| TEXAS INSTRUMENTS INCORPORATED
| Standard Linear and Logic Group
| IBIS Model of SN74LVCH16244A
| 16 Bit Buffer/Driver With 3 State Outputs
| This file contains package information for the following:
|  TSSOP 48-pin (DGG) package as [Component] LVCH16244A_DGG
|  SSOP 48-pin (DL) package as [Component] LVCH16244A_DL
| This device can be powered at the following Vccs:
|  3.3 volt Vcc
|  2.5 volt Vcc
|  1.8 volt Vcc
| This file provides unique models under the [Model Selector] for each Vcc.
| For operation at a specific Vcc, select the appropriate model after each
| [Model Selector] keyword.
[IBIS Ver]   3.2
[Comment char]  |_char
[File Name]   sn74lvch16244a.ibs
[File Rev]   1.1 | e_die
[Date]   March 8, 2002
[Source]   Data created from TI-SPICE simulations at TI-SLL.
[Notes]   The following is an IBIS list for the LVCH16244A.
   Please contact sllibis@ti.com with questions and
   comments concerning SLL IBIS models.
   - As there is no power clamp diode in the Input and I/O
   Models, we removed the Pwr Clamp table data from those Models.
   - Due to BUS-HOLD Circuit, there are non-monotonic
   warnings in I/O GND Clamp curve.
   -Due to the fact that the Device is 5-V Input/Output
   tolarent, the output model has some Non-Monotonic Warnings.
   - C_comp values are taken at a different test condition than
   the data sheet.
[Disclaimer] Property of Texas Instruments Incorporated.  Unauthorized
   reproduction and/or distribution is strictly prohibited.
   This product is protected under copyright law.
   Created  2001, (C) Copyright  2001, Texas Instruments
   Incorporated, All Rights Reserved
   UNLESS THERE IS A SIGNED, WRITTEN AGREEMENT TO THE
   CONTRARY, TEXAS INSTRUMENTS (TI) IS PROVIDING THE IBIS
   MODELS  AND WITHOUT ANY WARRANTY, EXPRESSED OR
   IMPLIED.  TI assumes no liability for:
   1) the accuracy of the IBIS models provided to your
   company;
   2) the proper functioning of these IBIS Models in your
   design or for any resulting applications; or
   3) infringement of patents, copyrights or intellectual
   property rights resulting from your use of these IBIS
   models.
   TI provides IBIS Models as a service to our customers.
   You and your company shall not distribute, sell or give
   these models to anyone else without prior written
   permission from TI.
   TI reserves the right to make changes to our products or
   to discontinue any semiconductor product or service
   without notice, and advises our customers to obtain the
   latest version of relevant information to verify, before
   placing orders, that the information being relied on is
   current.
   Please be aware that your receipt and use of the IBIS
   information provided shall serve as acceptance of these
   terms and conditions.  If you do not accept these terms,
   you should return or destroy the IBIS models and any
   other accompanying information immediately.
| Component LVCH16244A_DGG 48-pin TSSOP
[Component]   LVCH16244A_DGG
[Manufacturer]   Texas Instruments, Inc.
[Package]
|   typ   min   max
R_pkg   6.200e-02   5.000e-02   7.800e-02
L_pkg   3.527e-09   3.128e-09   4.255e-09
C_pkg   5.300e-13   4.170e-13   6.850e-13
[Pin]   signal_name   model_name   R_pin   L_pin   C_pin
1   1OE   LVCH16244A_OEIN   5.000e-02   4.250e-09   6.710e-13
2   1Y1   LVCH16244A_OUT   5.700e-02   3.956e-09   6.740e-13
3   1Y2   LVCH16244A_OUT   7.100e-02   3.922e-09   6.190e-13
4   GND   GND   7.800e-02   3.841e-09   6.180e-13
5   1Y3   LVCH16244A_OUT   5.600e-02   3.535e-09   5.550e-13
6   1Y4   LVCH16244A_OUT   5.800e-02   3.464e-09   5.030e-13
7   VCC   POWER   6.000e-02   3.362e-09   4.980e-13
8   2Y1   LVCH16244A_OUT   6.100e-02   3.293e-09   4.620e-13
9   2Y2   LVCH16244A_OUT   6.300e-02   3.240e-09   4.550e-13
10   GND   GND   6.300e-02   3.175e-09   4.420e-13
11   2Y3   LVCH16244A_OUT   6.400e-02   3.153e-09   4.290e-13
12   2Y4   LVCH16244A_OUT   6.500e-02   3.128e-09   4.180e-13
13   3Y1   LVCH16244A_OUT   6.500e-02   3.128e-09   4.180e-13
14   3Y2   LVCH16244A_OUT   6.400e-02   3.154e-09   4.290e-13
15   GND   GND   6.300e-02   3.174e-09   4.420e-13
16   3Y3   LVCH16244A_OUT   6.300e-02   3.241e-09   4.550e-13
17   3Y4   LVCH16244A_OUT   6.100e-02   3.293e-09   4.620e-13
18   VCC   POWER   6.000e-02   3.362e-09   4.970e-13
19   4Y1   LVCH16244A_OUT   5.800e-02   3.464e-09   5.030e-13
20   4Y2   LVCH16244A_OUT   5.600e-02   3.537e-09   5.600e-13
21   GND   GND   7.700e-02   3.839e-09   6.260e-13
22   4Y3   LVCH16244A_OUT   7.100e-02   3.917e-09   6.270e-13
23   4Y4   LVCH16244A_OUT   5.800e-02   3.955e-09   6.850e-13
24   4OE   LVCH16244A_OEIN   5.200e-02   4.255e-09   6.790e-13
25   3OE   LVCH16244A_OEIN   5.100e-02   4.254e-09   6.760e-13
26   4A4   LVCH16244A_IN   5.800e-02   3.957e-09   6.790e-13
27   4A3   LVCH16244A_IN   7.100e-02   3.920e-09   6.210e-13
28   GND   GND   7.800e-02   3.843e-09   6.220e-13
29   4A2   LVCH16244A_IN   5.600e-02   3.539e-09   5.600e-13
30   4A1   LVCH16244A_IN   5.800e-02   3.466e-09   5.030e-13
31   VCC   POWER   6.000e-02   3.363e-09   4.970e-13
32   3A4   LVCH16244A_IN   6.100e-02   3.294e-09   4.620e-13
33   3A3   LVCH16244A_IN   6.300e-02   3.241e-09   4.540e-13
34   GND   GND   6.300e-02   3.175e-09   4.410e-13
35   3A2   LVCH16244A_IN   6.400e-02   3.153e-09   4.290e-13
36   3A1   LVCH16244A_IN   6.500e-02   3.129e-09   4.170e-13
37   2A4   LVCH16244A_IN   6.500e-02   3.129e-09   4.170e-13
38   2A3   LVCH16244A_IN   6.400e-02   3.152e-09   4.290e-13
39   GND   GND   6.400e-02   3.176e-09   4.410e-13
40   2A2   LVCH16244A_IN   6.300e-02   3.241e-09   4.540e-13
41   2A1   LVCH16244A_IN   6.100e-02   3.293e-09   4.620e-13
42   VCC   POWER   6.000e-02   3.363e-09   4.970e-13
43   1A4   LVCH16244A_IN   5.800e-02   3.464e-09   5.030e-13
44   1A3   LVCH16244A_IN   5.600e-02   3.534e-09   5.610e-13
45   GND   GND   7.800e-02   3.841e-09   6.260e-13
46   1A2   LVCH16244A_IN   7.100e-02   3.920e-09   6.220e-13
47   1A1   LVCH16244A_IN   5.700e-02   3.955e-09   6.770e-13
48   2OE   LVCH16244A_OEIN   5.100e-02   4.252e-09   6.720e-13
| Component LVCH16244A_DL 48-pin SSOP
[Component]   LVCH16244A_DL
[Manufacturer]   Texas Instruments, Inc.
[Package]
|   typ   min   max
R_pkg   4.800e-02   3.800e-02   5.300e-02
L_pkg   6.046e-09   5.084e-09   7.968e-09
C_pkg   8.130e-13   5.690e-13   1.157e-12
[Pin]   signal_name   model_name   R_pin   L_pin   C_pin
1   1OE   LVCH16244A_OEIN   4.600e-02   7.968e-09   1.017e-12
2   1Y1   LVCH16244A_OUT   4.400e-02   7.299e-09   1.157e-12
3   1Y2   LVCH16244A_OUT   4.300e-02   6.765e-09   1.058e-12
4   GND   GND   4.100e-02   6.269e-09   9.330e-13
5   1Y3   LVCH16244A_OUT   3.800e-02   5.856e-09   8.290e-13
6   1Y4   LVCH16244A_OUT   4.600e-02   5.802e-09   7.900e-13
7   VCC   POWER   5.000e-02   5.656e-09   7.380e-13
8   2Y1   LVCH16244A_OUT   5.300e-02   5.500e-09   6.430e-13
9   2Y2   LVCH16244A_OUT   5.200e-02   5.304e-09   6.060e-13
10   GND   GND   5.300e-02   5.189e-09   5.830e-13
11   2Y3   LVCH16244A_OUT   5.100e-02   5.084e-09   5.690e-13
12   2Y4   LVCH16244A_OUT   5.300e-02   5.862e-09   8.330e-13
13   3Y1   LVCH16244A_OUT   5.300e-02   5.862e-09   8.330e-13
14   3Y2   LVCH16244A_OUT   5.100e-02   5.084e-09   5.690e-13
15   GND   GND   5.300e-02   5.189e-09   5.830e-13
16   3Y3   LVCH16244A_OUT   5.200e-02   5.304e-09   6.060e-13
17   3Y4   LVCH16244A_OUT   5.300e-02   5.500e-09   6.430e-13
18   VCC   POWER   5.000e-02   5.656e-09   7.380e-13
19   4Y1   LVCH16244A_OUT   4.600e-02   5.802e-09   7.900e-13
20   4Y2   LVCH16244A_OUT   3.800e-02   5.856e-09   8.290e-13
21   GND   GND   4.100e-02   6.269e-09   9.330e-13
22   4Y3   LVCH16244A_OUT   4.300e-02   6.765e-09   1.058e-12
23   4Y4   LVCH16244A_OUT   4.400e-02   7.299e-09   1.157e-12
24   4OE   LVCH16244A_OEIN   4.600e-02   7.968e-09   1.017e-12
25   3OE   LVCH16244A_OEIN   4.600e-02   7.968e-09   1.017e-12
26   4A4   LVCH16244A_IN   4.400e-02   7.299e-09   1.157e-12
27   4A3   LVCH16244A_IN   4.300e-02   6.765e-09   1.058e-12
28   GND   GND   4.100e-02   6.269e-09   9.330e-13
29   4A2   LVCH16244A_IN   3.800e-02   5.856e-09   8.290e-13
30   4A1   LVCH16244A_IN   4.600e-02   5.802e-09   7.900e-13
31   VCC   POWER   5.000e-02   5.656e-09   7.380e-13
32   3A4   LVCH16244A_IN   5.300e-02   5.500e-09   6.430e-13
33   3A3   LVCH16244A_IN   5.200e-02   5.304e-09   6.060e-13
34   GND   GND   5.300e-02   5.189e-09   5.830e-13
35   3A2   LVCH16244A_IN   5.100e-02   5.084e-09   5.690e-13
36   3A1   LVCH16244A_IN   5.300e-02   5.862e-09   8.330e-13
37   2A4   LVCH16244A_IN   5.300e-02   5.862e-09   8.330e-13
38   2A3   LVCH16244A_IN   5.100e-02   5.084e-09   5.690e-13
39   GND   GND   5.300e-02   5.189e-09   5.830e-13
40   2A2   LVCH16244A_IN   5.200e-02   5.304e-09   6.060e-13
41   2A1   LVCH16244A_IN   5.300e-02   5.500e-09   6.430e-13
42   VCC   POWER   5.000e-02   5.656e-09   7.380e-13
43   1A4   LVCH16244A_IN   4.600e-02   5.802e-09   7.900e-13
44   1A3   LVCH16244A_IN   3.800e-02   5.856e-09   8.290e-13
45   GND   GND   4.100e-02   6.269e-09   9.330e-13
46   1A2   LVCH16244A_IN   4.300e-02   6.765e-09   1.058e-12
47   1A1   LVCH16244A_IN   4.400e-02   7.299e-09   1.157e-12
48   2OE   LVCH16244A_OEIN   4.600e-02   7.967e-09   1.017e-12
|   Component   LVCH16244A_DGV   48-pin   TVSOP
[Component]   LVCH16244A_DGV
[Manufacturer]   Texas   Instruments,   Inc.
[Package]
|   typ   min   max
R_pkg   0.07   0.049   0.085
L_pkg   3.01E-09   2.74E-09   3.41E-09
C_pkg   3.71E-13   2.94E-13   5.11E-13
[Pin]   signal_name   model_name   R_pin   L_pin   C_pin
1   1OE   LVCH16244A_OEIN   0.049   3.39E-09   4.97E-13
2   1Y1   LVCH16244A_OUT   0.06   3.25E-09   5.02E-13
3   1Y2   LVCH16244A_OUT   0.077   3.31E-09   4.51E-13
4   GND   GND   0.085   3.3E-09   4.04E-13
5   1Y3   LVCH16244A_OUT   0.083   3.14E-09   3.6E-13
6   1Y4   LVCH16244A_OUT   0.077   3.02E-09   3.63E-13
7   VCC   POWER   0.065   2.88E-09   3.49E-13
8   2Y1   LVCH16244A_OUT   0.066   2.83E-09   3.14E-13
9   2Y2   LVCH16244A_OUT   0.067   2.8E-09   3.14E-13
10   GND   GND   0.069   2.75E-09   3.08E-13
11   2Y3   LVCH16244A_OUT   0.07   2.75E-09   3.01E-13
12   2Y4   LVCH16244A_OUT   0.071   2.75E-09   2.94E-13
13   3Y1   LVCH16244A_OUT   0.07   2.74E-09   2.94E-13
14   3Y2   LVCH16244A_OUT   0.07   2.75E-09   3.01E-13
15   GND   GND   0.069   2.75E-09   3.08E-13
16   3Y3   LVCH16244A_OUT   0.067   2.8E-09   3.14E-13
17   3Y4   LVCH16244A_OUT   0.066   2.83E-09   3.14E-13
18   VCC   POWER   0.065   2.88E-09   3.5E-13
19   4Y1   LVCH16244A_OUT   0.075   3.01E-09   3.63E-13
20   4Y2   LVCH16244A_OUT   0.08   3.13E-09   3.58E-13
21   GND   GND   0.084   3.3E-09   4.03E-13
22   4Y3   LVCH16244A_OUT   0.078   3.31E-09   4.52E-13
23   4Y4   LVCH16244A_OUT   0.062   3.26E-09   5.01E-13
24   4OE   LVCH16244A_OEIN   0.052   3.4E-09   4.96E-13
25   3OE   LVCH16244A_OEIN   0.053   3.4E-09   5.05E-13
26   4A4   LVCH16244A_IN   0.062   3.25E-09   5.11E-13
27   4A3   LVCH16244A_IN   0.077   3.31E-09   4.53E-13
28   GND   GND   0.082   3.29E-09   4.03E-13
29   4A2   LVCH16244A_IN   0.078   3.12E-09   3.59E-13
30   4A1   LVCH16244A_IN   0.074   3.01E-09   3.63E-13
31   VCC   POWER   0.065   2.88E-09   3.49E-13
32   3A4   LVCH16244A_IN   0.067   2.83E-09   3.14E-13
33   3A3   LVCH16244A_IN   0.067   2.8E-09   3.14E-13
34   GND   GND   0.069   2.75E-09   3.07E-13
35   3A2   LVCH16244A_IN   0.07   2.75E-09   3.01E-13
36   3A1   LVCH16244A_IN   0.07   2.74E-09   2.94E-13
37   2A4   LVCH16244A_IN   0.07   2.74E-09   2.94E-13
38   2A3   LVCH16244A_IN   0.07   2.75E-09   3.01E-13
39   GND   GND   0.069   2.75E-09   3.07E-13
40   2A2   LVCH16244A_IN   0.068   2.8E-09   3.14E-13
41   2A1   LVCH16244A_IN   0.067   2.83E-09   3.14E-13
42   VCC   POWER   0.064   2.88E-09   3.49E-13
43   1A4   LVCH16244A_IN   0.072   3E-09   3.62E-13
44   1A3   LVCH16244A_IN   0.078   3.12E-09   3.59E-13
45   GND   GND   0.084   3.3E-09   4.03E-13
46   1A2   LVCH16244A_IN   0.077   3.31E-09   4.51E-13
47   1A1   LVCH16244A_IN   0.062   3.26E-09   4.99E-13
48   2OE   LVCH16244A_OEIN   0.053   3.41E-09   4.94E-13
| Model LVCH16244A_IN
[Model Selector]   LVCH16244A_IN
LVCH16244A_IN_33   3.3 volt Vcc
LVCH16244A_IN_25   2.5 volt Vcc
LVCH16244A_IN_18   1.8 volt Vcc
| Model LVCH16244A_OEIN
[Model Selector]   LVCH16244A_OEIN
LVCH16244A_OEIN_33   3.3 volt Vcc
LVCH16244A_OEIN_25   2.5 volt Vcc
LVCH16244A_OEIN_18   1.8 volt Vcc
| Model LVCH16244A_OUT
[Model Selector]   LVCH16244A_OUT
LVCH16244A_OUT_33   3.3 volt Vcc
LVCH16244A_OUT_25   2.5 volt Vcc
LVCH16244A_OUT_18   1.8 volt Vcc
| Models and submodels in the file (9): LVCH16244A_IN_33 (Input), LVCH16244A_IN_25 (Input), LVCH16244A_IN_18 (Input), LVCH16244A_OEIN_33 (Input), LVCH16244A_OEIN_25 (Input), LVCH16244A_OEIN_18 (Input), LVCH16244A_OUT_33 (3-state), LVCH16244A_OUT_25 (3-state), LVCH16244A_OUT_18 (3-state)
